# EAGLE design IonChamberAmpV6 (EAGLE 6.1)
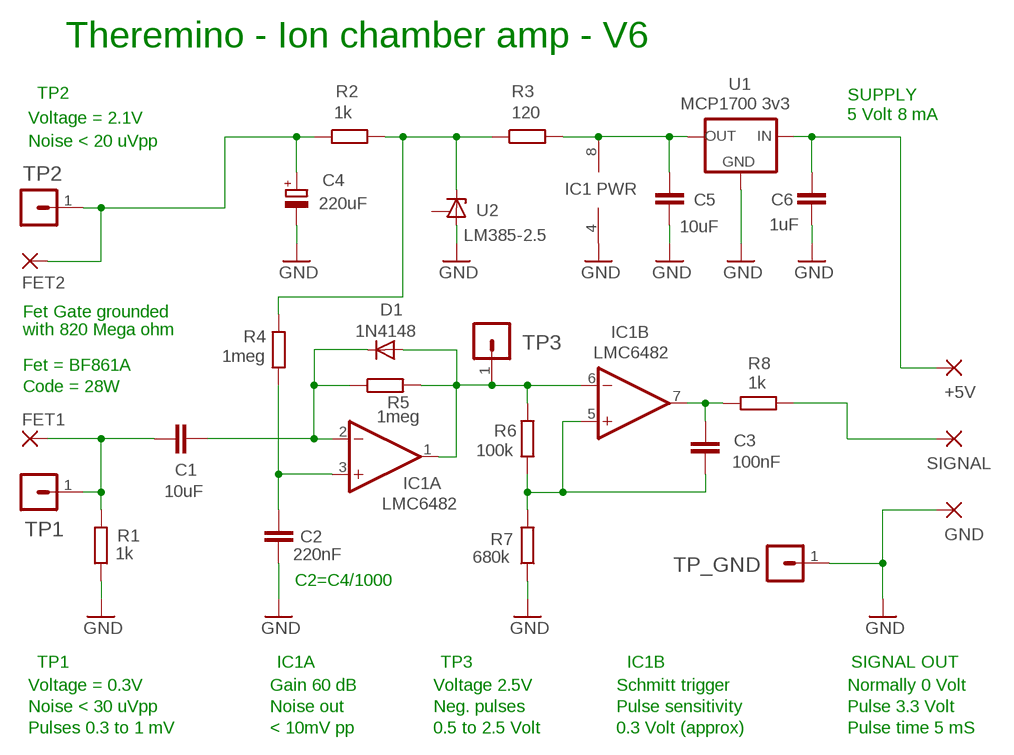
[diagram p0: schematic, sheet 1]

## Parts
+5V  WIREPAD1,6/0,8  [1,6/0,8]
C1  10uF  C-EUC0805  [C0805]
C2  220nF  C-EUC0805  [C0805]
C3  100nF  C-EUC0805  [C0805]
C4  220uF  CPOL-EUE2-5B  [E2-5B]
C5  10uF  C-EUC0805  [C0805]
C6  1uF  C-EUC0805  [C0805]
D1  1N4148  DIODE-SOD123  [SOD123]
FET1  WIREPADSMD1,90-2,54  [SMD1,90-2,54]
FET2  WIREPADSMD1,90-2,54  [SMD1,90-2,54]
GND  WIREPAD1,6/0,8  [1,6/0,8]
IC1  LMC6482  TL072P  [DIL08]
R1  1k  R-EU_R0805  [R0805]
R2  1k  R-EU_R0805  [R0805]
R3  120  R-EU_R0805  [R0805]
R4  1meg  R-EU_R1206_L  [R1206_L]
R5  1meg  R-EU_R0805  [R0805]
R6  100k  R-EU_R0805  [R0805]
R7  680k  R-EU_R0805  [R0805]
R8  1k  R-EU_R0805  [R0805]
SIGNAL  WIREPAD1,6/0,8  [1,6/0,8]
TP1  MA01-1  [MA01-1]
TP2  MA01-1  [MA01-1]
TP3  MA01-1  [MA01-1]
TP_GND  MA01-1  [MA01-1]
U1  MCP1700 3v3  MCP1700SOT23L  [SOT23_L]
U2  LM385-2.5  LM3851  [TO92L1]

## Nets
GND: C2.1 C4.- C5.2 C6.2 GND.1(P) IC1.4(P:V-) R1.1 R7.1 TP_GND.1 U1.1(GND) U2.1(A)
N$1: C3.2 IC1.5(B:+IN) R6.1 R7.2
N$2: C2.2 IC1.3(A:+IN) R4.1
N$3: D1.A IC1.1(A:OUT) IC1.6(B:-IN) R5.2 R6.2 TP3.1
N$5: C3.1 IC1.7(B:OUT) R8.1
N$6: C1.2 FET1.1(P) R1.2 TP1.1
N$7: R8.2 SIGNAL.1(P)
N$8: +5V.1(P) C6.1 U1.3(IN)
N$9: C5.1 IC1.8(P:V+) R3.2 U1.2(OUT)
N$10: R2.2 R3.1 R4.2 U2.2(C)
N$11: C1.1 D1.C IC1.2(A:-IN) R5.1
TP2: C4.+ FET2.1(P) R2.1 TP2.1
Unconnected: U2.3(NC)

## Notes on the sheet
- Theremino - Ion chamber amp - V6
- TP2 | SUPPLY
- Voltage = 2.1V | 5 Volt 8 mA
- Noise < 20 uVpp
- IC1 PWR
- Fet Gate grounded
- with 820 Mega ohm
- Fet = BF861A
- Code = 28W
- C2=C4/1000
- TP1 | IC1A | TP3 | IC1B | SIGNAL OUT
- Voltage = 0.3V | Gain 60 dB | Voltage 2.5V | Schmitt trigger | Normally 0 Volt
- Noise < 30 uVpp | Noise out | Neg. pulses | Pulse sensitivity | Pulse 3.3 Volt
- Pulses 0.3 to 1 mV | < 10mV pp | 0.5 to 2.5 Volt | 0.3 Volt (approx) | Pulse time 5 mS

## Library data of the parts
+5V FET1 FET2 GND SIGNAL = 00-LIVIO:WIREPAD: Wire PAD connect wire on PCB
C1-C3 C5 C6 = 00-LIVIO:C-EU: CAPACITOR, European symbol
C4 = 00-LIVIO:CPOL-EU: POLARIZED CAPACITOR, European symbol
D1 = 00-LIVIO:DIODE-: DIODE
IC1 = linear:TL072: OP AMP
R1-R8 = 00-LIVIO:R-EU_: RESISTOR, European symbol
TP1-TP3 TP_GND = 03-con-lstb-M:MA01-1: PIN HEADER
U1 = 00-LIVIO:MCP1700: Linear regulator Quescient courrent 1.8uA Input 2.3v to 6v Output 1.2v 1.8v 2.5v 3.0v 3.3v 5.0v
U2 = 00-LIVIO:LM385: LM385 Shunt regulator (1.2 or 2.5 Volt) pin compatible with LM4040, more precise (2.048 / 2.5 / 3.0 / 8.192 and 10 Volt)

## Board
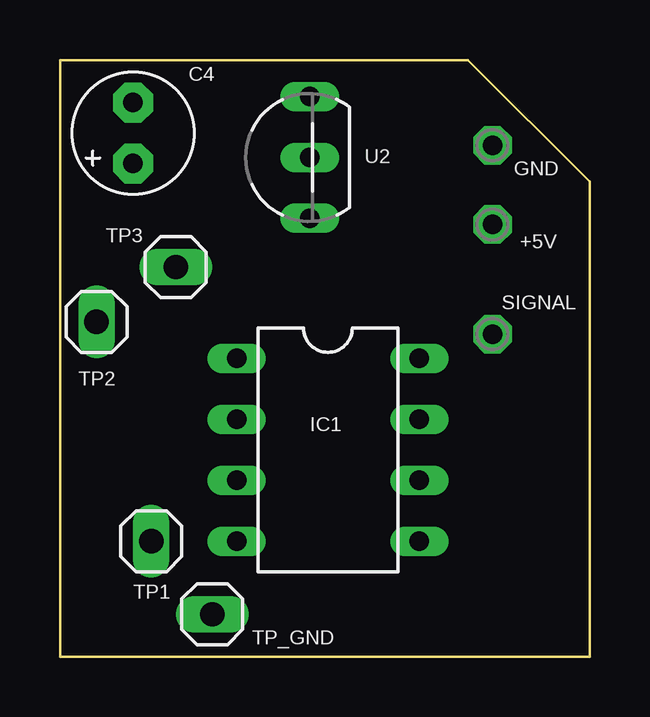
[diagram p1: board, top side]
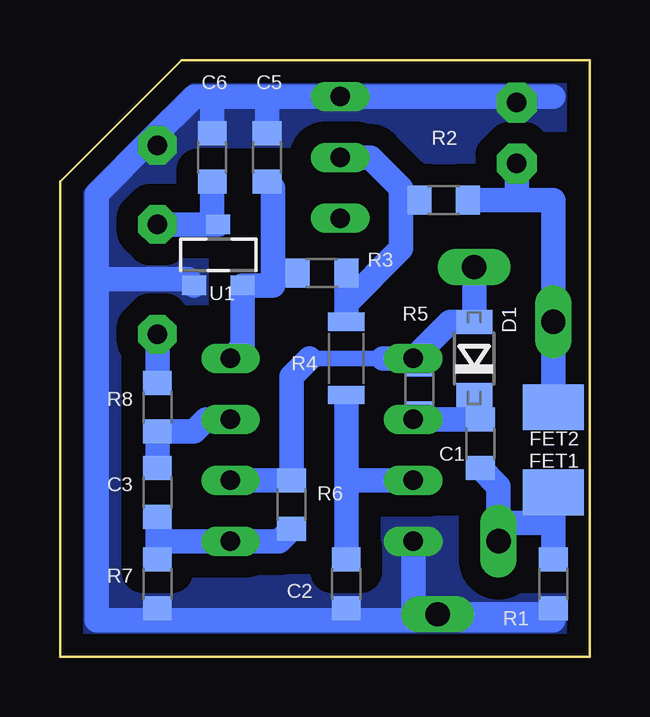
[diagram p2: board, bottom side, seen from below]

Size 22.1 x 24.89 mm. Coordinates in mm from the lower left corner, seen from the top.
Outline: 0,0 22.1,0 22.1,19.81 17.02,24.89 0,24.89 0,0
Copper layers (1*16): Top 0.035mm / dielectric 1.5mm / Bottom 0.035mm
Design rules: minimum track width 10mil, minimum drill 0.6mm, track to track 8mil, track to pad 8mil, pad to pad 8mil, via to via 8mil, smd to smd 8mil, copper to edge 31mil, drill to drill 8mil, minimum pad ring 5mil, minimum via ring 8mil, stop-mask expansion 4mil, vias tented up to drill 0mil, thermal gap 47mil

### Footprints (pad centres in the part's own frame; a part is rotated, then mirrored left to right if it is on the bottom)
1,6/0,8 = drill 0.813 pad 1.6 octagon: 1 0,0
C0805 = smd 1 x 1.2: 1 -1.016,0; 2 1.016,0
E2-5B = drill 0.813 pad 1.676 octagon: + -1.27,0; - 1.27,0
SOD123 = smd 1 x 1.5: A 1.524,0; C -1.524,0
SMD1,90-2,54 = smd 1.905 x 2.54: 1 0,0
DIL08 = drill 0.813 long: 1 -3.81,-3.81; 2 -1.27,-3.81; 3 1.27,-3.81; 4 3.81,-3.81; 5 3.81,3.81; 6 1.27,3.81; 7 -1.27,3.81; 8 -3.81,3.81
R0805 = smd 1 x 1.2: 1 -1.016,0; 2 1.016,0
R1206_L = smd 0.762 x 1.524: 1 -1.524,0; 2 1.524,0
MA01-1 = drill 1.016 long: 1 0,0
SOT23_L = smd 1 x 0.8: 1 -1.016,-1.27; 2 1.016,-1.27; 3 0,1.27
TO92L1 = drill 0.813 long: 1 2.54,0; 2 0,0; 3 -2.54,0

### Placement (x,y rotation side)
+5V  18.03,18.03 0 top
C1  4.57,8.89 270 bottom
C2  10.16,3.05 90 bottom
C3  18.03,6.86 270 bottom
C4  3.05,21.84 90 top
C5  13.46,20.83 90 bottom
C6  15.75,20.83 90 bottom
D1  4.83,12.45 90 bottom
FET1  1.52,6.86 90 bottom
FET2  1.52,10.41 270 bottom
GND  18.03,21.34 0 top
IC1  11.18,8.64 270 top
R1  1.52,3.05 90 bottom
R2  6.1,19.05 180 bottom
R3  11.18,16 180 bottom
R4  10.16,12.45 90 bottom
R5  7.11,11.18 90 bottom
R6  12.45,6.35 90 bottom
R7  18.03,3.05 90 bottom
R8  18.03,10.41 90 bottom
SIGNAL  18.03,13.46 0 top
TP1  3.81,4.83 180 top
TP2  1.52,13.97 0 top
TP3  4.83,16.26 90 top
TP_GND  6.35,1.78 90 top
U1  15.49,16.76 0 bottom
U2  10.41,20.83 90 top

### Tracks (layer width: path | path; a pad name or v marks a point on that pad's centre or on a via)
GND
  Bottom 1.016: 6.35,1.52 1.52,1.52 1.52,1.78 | 10.16,1.52 18.03,1.52 | 18.03,1.52 20.57,1.52 20.57,15.75 | 10.16,1.52 6.35,1.52 | 6.35,1.52 TP_GND.1 | TP_GND.1 7.37,1.78 IC1.4 | 3.05,23.37 1.52,23.37 | C2.1 10.16,1.52 | U1.1 16.76,15.75 20.57,15.75 | R1.1 1.52,1.78 | R7.1 18.03,1.52 | 3.05,23.37 C4.- | 13.46,23.37 U2.1 3.05,23.37 | 13.46,23.37 15.75,23.37 | 15.75,23.37 16.51,23.37 18.29,21.59 | 18.29,21.59 20.57,19.3 20.57,15.75 | GND.1 18.29,21.59 | TP_GND.1 1.52,1.78 | C5.2 13.46,23.37 | C6.2 15.75,23.37
  pour Bottom (isolate 0.9, rank 6, no thermals): -1,-1 23.1,-1 23.1,25.89 -1,25.89
N$1
  Bottom 1.016: R6.1 12.95,4.83 IC1.5 18.03,4.83 | R7.2 18.03,4.83 | 18.03,4.83 C3.2
N$2
  Bottom 0.6: 10.16,10.67 R4.1
  Bottom 1.016: C2.2 10.16,7.37 | IC1.3 10.16,7.37 | 10.16,7.37 10.16,10.67
N$3
  Bottom 0.65: 8.64,12.45 11.68,12.45
  Bottom 1.016: IC1.1 5.84,13.97 D1.A TP3.1 | IC1.1 8.64,12.45 | 11.68,12.45 12.45,11.68 R6.2 IC1.6 | R5.2 7.37,12.19 IC1.1
N$5
  Bottom 1.016: C3.1 R8.1 16.51,9.4 16,9.91 IC1.7
N$6
  Bottom 1.016: 1.52,5.59 3.81,5.59 | 3.81,5.59 3.81,7.11 C1.2 | 1.52,5.59 FET1.1 | R1.2 1.52,5.59 | TP1.1 3.81,5.59
N$7
  Bottom 1.016: SIGNAL.1 R8.2
N$8
  Bottom 1.016: 15.75,18.03 +5V.1 | U1.3 15.75,18.03 | 15.75,18.03 C6.1
N$9
  Bottom 1.016: IC1.8 14.48,12.95 U1.2 13.21,15.49 13.21,16 | C5.1 13.21,19.56 13.21,16 | R3.2 13.21,16
N$10
  Bottom 0.6: 10.16,14.22 R4.2
  Bottom 1.016: 10.16,14.73 10.16,14.22 | 10.16,14.73 7.87,17.02 7.87,19.05 | R2.2 7.87,19.05 | U2.2 9.14,20.83 7.87,19.56 7.87,19.05 | 10.16,14.73 R3.1
N$11
  Bottom 1.016: D1.C 4.57,10.92 C1.1 IC1.2 7.37,10.16 R5.1
TP2
  Bottom 1.016: FET2.1 TP2.1 1.52,19.05 3.05,19.05 | 3.05,19.05 R2.1 | C4.+ 3.05,19.05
